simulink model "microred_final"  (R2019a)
settings: Solver=VariableStepAuto  StartTime=0.0  StopTime=24*60*60  FixedStep=1  RelTol=1e-3
undefined symbols (not defined in the file): A, B, C, cargagenerador, CoeficienteProduccion, Consumo_valores, consumogenerador, D1, Dd, Delta, irradiancia_valores, j, magnitude, PotenciaAerogenerador, precioelectricidad_valores, Precioventaelectricidad, Tiempo, VelocidadAerogenerador, viento_valores
libraries: powerlib x42, powerlib_meascontrol x6
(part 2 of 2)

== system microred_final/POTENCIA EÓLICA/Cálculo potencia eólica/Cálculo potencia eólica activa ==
  Perfil de viento : Inport
  " Coeficiente de potencia" : Subsystem
  Curva de Producción : Lookup_n-D  NumberOfTableDimensions=1  BreakpointsForDimension1=VelocidadAerogenerador  Table=PotenciaAerogenerador  InternalRulePriority=Speed  RndMeth=Simplest
  Modo Trabajo : Constant  Value=Modo
  Número de Aerogeneradores : Gain  Gain=NumAerogeneradores
  Scope3 : Scope
  Scope4 : Scope
  Switch : Switch  Criteria=u2 > Threshold  Threshold=1.5
  km/h --> m/s : Gain  Gain=1000/3600
  Potencia eólica activa : Outport
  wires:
  Perfil de viento/1 -> km/h --> m/s/1
  Switch/1 -> Número de Aerogeneradores/1
  km/h --> m/s/1 -> Curva de Producción/1, " Coeficiente de potencia"/1(m/s)
  Curva de Producción/1 -> Scope4/1, Switch/3
  Modo Trabajo/1 -> Switch/2
  " Coeficiente de potencia"/1(Potencia) -> Scope3/1, Switch/1
  Número de Aerogeneradores/1 -> Potencia eólica activa/1

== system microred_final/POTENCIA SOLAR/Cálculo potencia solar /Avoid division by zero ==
  I : Inport
  Complex to Magnitude-Angle : ComplexToMagnitudeAngle
  Magnitude-Angle to Complex : MagnitudeAngleToComplex
  Saturation1 : Saturate  UpperLimit=inf  LowerLimit=1e-6
  O : Outport
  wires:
  Complex to Magnitude-Angle/2 -> Magnitude-Angle to Complex/2
  Magnitude-Angle to Complex/1 -> O/1
  Complex to Magnitude-Angle/1 -> Saturation1/1
  Saturation1/1 -> Magnitude-Angle to Complex/1
  I/1 -> Complex to Magnitude-Angle/1

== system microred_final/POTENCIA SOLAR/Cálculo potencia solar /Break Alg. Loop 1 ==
  In : Inport
  Complex to Real-Imag : ComplexToRealImag
  Real-Imag to Complex : RealImagToComplex
  imag : Subsystem  mask(Transfer Function with Initial Outputs){N=[1], D=[0.1 1], Y0=0, U0=0}
      mask prompts: N "Numerator:"; D "Denominator:"; Y0 "Initial output:"; U0 "Initial input:"
      mask help: Vector expressions for numerator, and denominator. Coefficients are in descending powers of s.
      mask init:
      | [A,B,C,Dd]=tf2ss(N,D);if (isempty(Y0));[m,n]=size(A);X0=zeros(1,m); end; if (isempty(U0));[m,p]=size(B);U0=zeros(1,p);end;X0=getxo(A,B,C,Dd,U0,Y0,0);
  real : Subsystem  mask(Transfer Function with Initial Outputs){N=[1], D=[0.1 1], Y0=0, U0=0}
      mask prompts: N "Numerator:"; D "Denominator:"; Y0 "Initial output:"; U0 "Initial input:"
      mask help: Vector expressions for numerator, and denominator. Coefficients are in descending powers of s.
      mask init:
      | [A,B,C,Dd]=tf2ss(N,D);if (isempty(Y0));[m,n]=size(A);X0=zeros(1,m); end; if (isempty(U0));[m,p]=size(B);U0=zeros(1,p);end;X0=getxo(A,B,C,Dd,U0,Y0,0);
  Out : Outport
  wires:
  Complex to Real-Imag/1 -> real/1(In1)
  Complex to Real-Imag/2 -> imag/1(In1)
  In/1 -> Complex to Real-Imag/1
  Real-Imag to Complex/1 -> Out/1
  real/1(Out1) -> Real-Imag to Complex/1
  imag/1(Out1) -> Real-Imag to Complex/2

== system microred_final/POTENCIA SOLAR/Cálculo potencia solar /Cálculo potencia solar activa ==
  Perfil de irradiancia : Inport
  Area de cada panel solar : Constant  Value=AreaPanel
  Número de paneles solares : Gain  Gain=NumPaneles
  Psolar= irradiancia*area*eficiencia : Product  Inputs=3
  Rendimiento de los paneles solares : Constant  Value=RendimientoPanel/100
  "Potencia solar activa " : Outport
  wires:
  Perfil de irradiancia/1 -> Psolar= irradiancia*area*eficiencia/1
  Psolar= irradiancia*area*eficiencia/1 -> Número de paneles solares/1
  Rendimiento de los paneles solares/1 -> Psolar= irradiancia*area*eficiencia/3
  Area de cada panel solar/1 -> Psolar= irradiancia*area*eficiencia/2
  Número de paneles solares/1 -> "Potencia solar activa "/1

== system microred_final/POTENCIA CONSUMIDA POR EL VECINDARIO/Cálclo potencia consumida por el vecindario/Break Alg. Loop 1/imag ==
  In1 : Inport
  State Space : StateSpace  A=A  B=B  C=C  D=Dd  InitialCondition=X0
  Out1 : Outport  InitialOutput=0
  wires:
  State Space/1 -> Out1/1
  In1/1 -> State Space/1

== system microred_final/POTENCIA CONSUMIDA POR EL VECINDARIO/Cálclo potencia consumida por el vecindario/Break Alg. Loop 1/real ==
  In1 : Inport
  State Space : StateSpace  A=A  B=B  C=C  D=Dd  InitialCondition=X0
  Out1 : Outport  InitialOutput=0
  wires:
  State Space/1 -> Out1/1
  In1/1 -> State Space/1

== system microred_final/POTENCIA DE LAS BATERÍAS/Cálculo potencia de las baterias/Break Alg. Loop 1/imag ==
  In1 : Inport
  State Space : StateSpace  A=A  B=B  C=C  D=Dd  InitialCondition=X0
  Out1 : Outport  InitialOutput=0
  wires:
  State Space/1 -> Out1/1
  In1/1 -> State Space/1

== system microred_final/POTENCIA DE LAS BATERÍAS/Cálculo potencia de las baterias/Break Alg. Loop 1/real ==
  In1 : Inport
  State Space : StateSpace  A=A  B=B  C=C  D=Dd  InitialCondition=X0
  Out1 : Outport  InitialOutput=0
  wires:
  State Space/1 -> Out1/1
  In1/1 -> State Space/1

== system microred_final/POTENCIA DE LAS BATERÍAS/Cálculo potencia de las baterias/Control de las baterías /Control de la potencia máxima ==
  Constant : Constant  Value=ModoEnergetico
  Dot Product : DotProduct
  Modo disponibilidad : Subsystem  mask{CargaBaterias=60}
      mask prompts: CargaBaterias "Porcentaje de carga de las baterias (%)"
  Modo isla o optimizacion de la energía : Subsystem
  Potencia máxima : Scope
  Prioridad vender a la red : Subsystem  mask{Pventa=38, Pcompra=0.093}
      mask prompts: Pventa "Precio de venta (€/MWh)"; Pcompra "Precio de compra (€/KWh)"
  Signo de la potencia : Switch  Criteria=u2 > Threshold  Threshold=1
  Signo de la potencia1 : Switch  Criteria=u2 > Threshold  Threshold=2
  "Potencia máxima " : Outport
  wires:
  Constant/1 -> Dot Product/1
  [ModoMicrorred] -> Dot Product/2
  Dot Product/1 -> Signo de la potencia1/2, Signo de la potencia/2
  Signo de la potencia1/1 -> Signo de la potencia/1
  Modo isla o optimizacion de la energía/1("Potencia máxima ") -> Signo de la potencia/3
  Modo disponibilidad/1("Potencia máxima ") -> Signo de la potencia1/1
  Prioridad vender a la red/1("Potencia máxima ") -> Signo de la potencia1/3
  Signo de la potencia/1 -> Potencia máxima/1, "Potencia máxima "/1  "Potencia  máxima en w"

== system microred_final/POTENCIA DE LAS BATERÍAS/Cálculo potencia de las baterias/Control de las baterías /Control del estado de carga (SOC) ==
  Potencia máxima : Inport
  Potencia si supero limites : Constant  Value=0
  Potencia si supero limites1 : Constant  Value=0
  SOC INFERIOR : Switch  Threshold=L_Inf
  SOC SUPERIOR : Switch  Threshold=L_Sup
  Si va a aumentar el SOC : Switch
  Si va a bajar el SOC : Switch
  Potencia de las baterias : Outport
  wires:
  Si va a aumentar el SOC/1 -> SOC INFERIOR/3
  Si va a bajar el SOC/1 -> SOC SUPERIOR/1
  SOC INFERIOR/1 -> Potencia de las baterias/1
  SOC SUPERIOR/1 -> SOC INFERIOR/1
  Potencia máxima/1 -> SOC SUPERIOR/3, Si va a aumentar el SOC/2, Si va a aumentar el SOC/1, Si va a bajar el SOC/2, Si va a bajar el SOC/3
  [SOC] -> SOC INFERIOR/2
  [SOC] -> SOC SUPERIOR/2
  Potencia si supero limites/1 -> Si va a bajar el SOC/1
  Potencia si supero limites1/1 -> Si va a aumentar el SOC/3

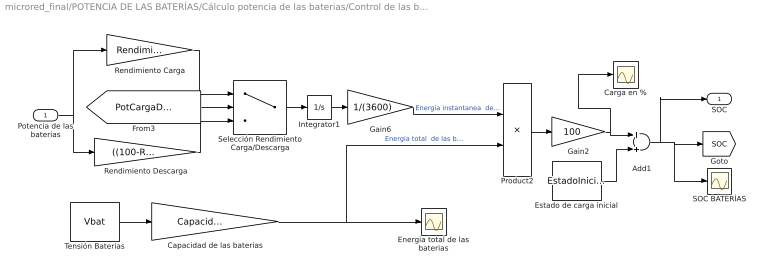
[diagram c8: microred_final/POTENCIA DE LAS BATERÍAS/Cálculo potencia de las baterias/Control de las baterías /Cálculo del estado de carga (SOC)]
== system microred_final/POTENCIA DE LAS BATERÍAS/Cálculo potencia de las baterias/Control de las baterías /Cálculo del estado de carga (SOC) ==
  Potencia de las baterias : Inport
  Add1 : Sum
  Capacidad de las baterias : Gain  Gain=Capacidad
  Carga en % : Scope
  Energia total de las baterias : Scope
  Estado de carga inicial : Constant  Value=EstadoInicial
  Gain2 : Gain  Gain=100
  Gain6 : Gain  Gain=1/(3600)
  Integrator1 : Integrator
  Product2 : Product  Inputs=*/
  Rendimiento Carga : Gain  Gain=Rendimiento/100
  Rendimiento Descarga : Gain  Gain=((100-Rendimiento)+100)/100
  SOC BATERÍAS : Scope
  Selección Rendimiento Carga/Descarga : Switch
  Tensión Baterias : Constant  Value=Vbat
  SOC : Outport
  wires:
  [PotCargaDescarga] -> Selección Rendimiento Carga/Descarga/2
  Estado de carga inicial/1 -> Add1/2
  Add1/1 -> SOC/1, [SOC], SOC BATERÍAS/1
  Product2/1 -> Gain2/1
  Rendimiento Carga/1 -> Selección Rendimiento Carga/Descarga/1
  Selección Rendimiento Carga/Descarga/1 -> Integrator1/1
  Gain6/1 -> Product2/1  "Energia instantanea  de las baterias"
  Rendimiento Descarga/1 -> Selección Rendimiento Carga/Descarga/3
  Tensión Baterias/1 -> Capacidad de las baterias/1
  Integrator1/1 -> Gain6/1
  Gain2/1 -> Add1/1, Carga en %/1
  Potencia de las baterias/1 -> Rendimiento Carga/1, Rendimiento Descarga/1
  Capacidad de las baterias/1 -> Product2/2, Energia total de las baterias/1  "Energia total  de las baterias"

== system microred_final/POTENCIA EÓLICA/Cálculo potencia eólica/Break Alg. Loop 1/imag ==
  In1 : Inport
  State Space : StateSpace  A=A  B=B  C=C  D=Dd  InitialCondition=X0
  Out1 : Outport  InitialOutput=0
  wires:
  State Space/1 -> Out1/1
  In1/1 -> State Space/1

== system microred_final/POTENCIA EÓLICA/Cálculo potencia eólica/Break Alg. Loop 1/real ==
  In1 : Inport
  State Space : StateSpace  A=A  B=B  C=C  D=Dd  InitialCondition=X0
  Out1 : Outport  InitialOutput=0
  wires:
  State Space/1 -> Out1/1
  In1/1 -> State Space/1

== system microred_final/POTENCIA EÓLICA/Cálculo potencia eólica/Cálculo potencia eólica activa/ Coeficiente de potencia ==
  m/s : Inport
  " " : Constant  Value=3
  1/2 : Constant  Value=1/2
  "Curva coficiente de produción " : Lookup_n-D  NumberOfTableDimensions=1  BreakpointsForDimension1=VelocidadAerogenerador  Table=CoeficienteProduccion  InternalRulePriority=Speed  RndMeth=Simplest
  Densidad del viento : Constant  Value=Densidad
  "Peólica(total)=1/2(p*A*V^3) " : Product  Inputs=4
  Peólica=1/2(p*A*V^3)*Cp : Product
  Square : Math  Operator=pow
  Superficie de viento que incide en las aspas : Constant  Value=SupViento
  Potencia : Outport
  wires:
  "Curva coficiente de produción "/1 -> Peólica=1/2(p*A*V^3)*Cp/1
  m/s/1 -> Square/1, "Curva coficiente de produción "/1
  Square/1 -> "Peólica(total)=1/2(p*A*V^3) "/2
  Densidad del viento/1 -> "Peólica(total)=1/2(p*A*V^3) "/3
  "Peólica(total)=1/2(p*A*V^3) "/1 -> Peólica=1/2(p*A*V^3)*Cp/2
  Peólica=1/2(p*A*V^3)*Cp/1 -> Potencia/1
  Superficie de viento que incide en las aspas/1 -> "Peólica(total)=1/2(p*A*V^3) "/4
  1/2/1 -> "Peólica(total)=1/2(p*A*V^3) "/1
  " "/1 -> Square/2

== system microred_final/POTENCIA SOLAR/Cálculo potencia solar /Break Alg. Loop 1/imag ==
  In1 : Inport
  State Space : StateSpace  A=A  B=B  C=C  D=Dd  InitialCondition=X0
  Out1 : Outport  InitialOutput=0
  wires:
  State Space/1 -> Out1/1
  In1/1 -> State Space/1

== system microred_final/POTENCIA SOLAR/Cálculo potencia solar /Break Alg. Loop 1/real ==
  In1 : Inport
  State Space : StateSpace  A=A  B=B  C=C  D=Dd  InitialCondition=X0
  Out1 : Outport  InitialOutput=0
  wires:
  State Space/1 -> Out1/1
  In1/1 -> State Space/1

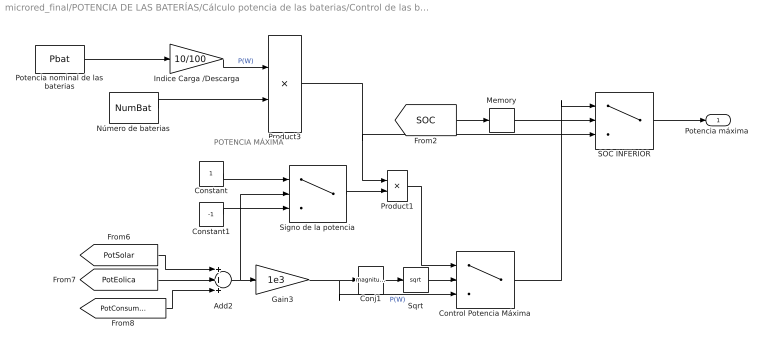
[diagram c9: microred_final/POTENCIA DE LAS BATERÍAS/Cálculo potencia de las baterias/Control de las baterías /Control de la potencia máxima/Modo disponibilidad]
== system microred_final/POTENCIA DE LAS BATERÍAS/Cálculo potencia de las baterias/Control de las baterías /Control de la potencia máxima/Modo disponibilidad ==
  note: POTENCIA MÁXIMA
  Add2 : Sum  Inputs=+++
  Conj1 : Math  Operator=magnitude^2
  Constant : Constant
  Constant1 : Constant  Value=-1
  Control Potencia Máxima : Switch  Criteria=u2 > Threshold  Threshold=(Pbat*NumBat)*(10/100)
  Gain3 : Gain  Gain=1e3
  Indice Carga /Descarga : Gain  Gain=10/100
  Memory : Memory  InheritSampleTime=on  LinearizeMemory=on  LinearizeAsDelay=on
  Número de baterias : Constant  Value=NumBat
  Potencia nominal de las baterias : Constant  Value=Pbat
  Product1 : Product  Inputs=**
  Product3 : Product  Inputs=**
  SOC INFERIOR : Switch  Threshold=CargaBaterias  ZeroCross=off
  Signo de la potencia : Switch
  Sqrt : Sqrt
  "Potencia máxima " : Outport
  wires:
  Potencia nominal de las baterias/1 -> Indice Carga /Descarga/1
  Constant1/1 -> Signo de la potencia/3
  Product3/1 -> Product1/1, SOC INFERIOR/3
  Signo de la potencia/1 -> Product1/2
  Constant/1 -> Signo de la potencia/1
  Conj1/1 -> Sqrt/1
  Product1/1 -> Control Potencia Máxima/1
  [PotEolica] -> Add2/2
  [PotConsumida] -> Add2/3
  Add2/1 -> Gain3/1, Signo de la potencia/2
  [PotSolar] -> Add2/1
  Indice Carga /Descarga/1 -> Product3/1  "P(W)"
  Número de baterias/1 -> Product3/2
  Gain3/1 -> Conj1/1, Control Potencia Máxima/3  "P(W)"
  Sqrt/1 -> Control Potencia Máxima/2
  Control Potencia Máxima/1 -> SOC INFERIOR/1
  SOC INFERIOR/1 -> "Potencia máxima "/1
  [SOC] -> Memory/1
  Memory/1 -> SOC INFERIOR/2

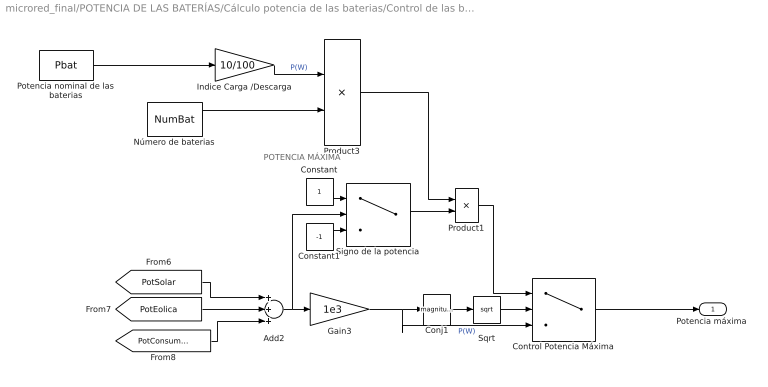
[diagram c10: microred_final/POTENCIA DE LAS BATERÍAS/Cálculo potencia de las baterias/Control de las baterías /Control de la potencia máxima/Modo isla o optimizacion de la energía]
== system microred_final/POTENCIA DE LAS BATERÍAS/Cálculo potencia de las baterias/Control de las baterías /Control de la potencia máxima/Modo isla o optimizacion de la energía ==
  note: POTENCIA MÁXIMA
  Add2 : Sum  Inputs=+++
  Conj1 : Math  Operator=magnitude^2
  Constant : Constant
  Constant1 : Constant  Value=-1
  Control Potencia Máxima : Switch  Criteria=u2 > Threshold  Threshold=(Pbat*NumBat)*(10/100)
  Gain3 : Gain  Gain=1e3
  Indice Carga /Descarga : Gain  Gain=10/100
  Número de baterias : Constant  Value=NumBat
  Potencia nominal de las baterias : Constant  Value=Pbat
  Product1 : Product  Inputs=**
  Product3 : Product  Inputs=**
  Signo de la potencia : Switch
  Sqrt : Sqrt
  "Potencia máxima " : Outport
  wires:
  Control Potencia Máxima/1 -> "Potencia máxima "/1
  Sqrt/1 -> Control Potencia Máxima/2
  Gain3/1 -> Control Potencia Máxima/3, Conj1/1  "P(W)"
  Número de baterias/1 -> Product3/2
  Indice Carga /Descarga/1 -> Product3/1  "P(W)"
  [PotSolar] -> Add2/1
  Add2/1 -> Signo de la potencia/2, Gain3/1
  [PotConsumida] -> Add2/3
  [PotEolica] -> Add2/2
  Product1/1 -> Control Potencia Máxima/1
  Conj1/1 -> Sqrt/1
  Constant/1 -> Signo de la potencia/1
  Signo de la potencia/1 -> Product1/2
  Product3/1 -> Product1/1
  Constant1/1 -> Signo de la potencia/3
  Potencia nominal de las baterias/1 -> Indice Carga /Descarga/1

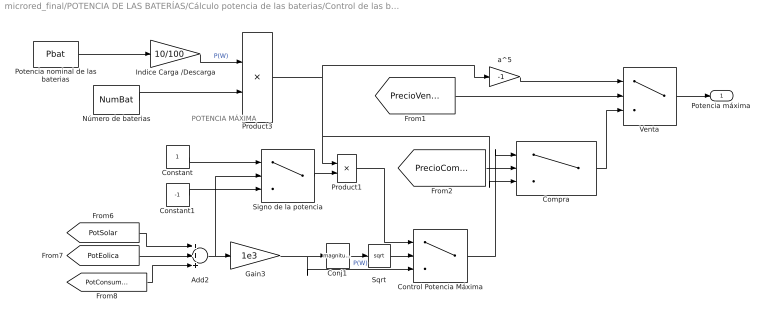
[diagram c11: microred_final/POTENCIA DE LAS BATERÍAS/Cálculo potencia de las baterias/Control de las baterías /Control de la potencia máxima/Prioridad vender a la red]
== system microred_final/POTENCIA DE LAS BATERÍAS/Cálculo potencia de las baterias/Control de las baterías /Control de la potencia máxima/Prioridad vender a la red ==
  note: POTENCIA MÁXIMA
  Add2 : Sum  Inputs=+++
  Compra : Switch  Threshold=Pcompra  ZeroCross=off
  Conj1 : Math  Operator=magnitude^2
  Constant : Constant
  Constant1 : Constant  Value=-1
  Control Potencia Máxima : Switch  Criteria=u2 > Threshold  Threshold=(Pbat*NumBat)*(10/100)
  Gain3 : Gain  Gain=1e3
  Indice Carga /Descarga : Gain  Gain=10/100
  Número de baterias : Constant  Value=NumBat
  Potencia nominal de las baterias : Constant  Value=Pbat
  Product1 : Product  Inputs=**
  Product3 : Product  Inputs=**
  Signo de la potencia : Switch
  Sqrt : Sqrt
  Venta : Switch  Threshold=Pventa  ZeroCross=off
  a^5 : Gain  Gain=-1
  "Potencia máxima " : Outport
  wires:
  [PrecioVenta] -> Venta/2
  Venta/1 -> "Potencia máxima "/1
  Control Potencia Máxima/1 -> Compra/1
  Sqrt/1 -> Control Potencia Máxima/2
  Gain3/1 -> Control Potencia Máxima/3, Conj1/1  "P(W)"
  Número de baterias/1 -> Product3/2
  Indice Carga /Descarga/1 -> Product3/1  "P(W)"
  [PotSolar] -> Add2/1
  Add2/1 -> Signo de la potencia/2, Gain3/1
  [PotConsumida] -> Add2/3
  [PotEolica] -> Add2/2
  Product1/1 -> Control Potencia Máxima/1
  Conj1/1 -> Sqrt/1
  Constant/1 -> Signo de la potencia/1
  Signo de la potencia/1 -> Product1/2
  Product3/1 -> a^5/1, Compra/3, Product1/1
  Constant1/1 -> Signo de la potencia/3
  Potencia nominal de las baterias/1 -> Indice Carga /Descarga/1
  [PrecioCompra] -> Compra/2
  a^5/1 -> Venta/1
  Compra/1 -> Venta/3
